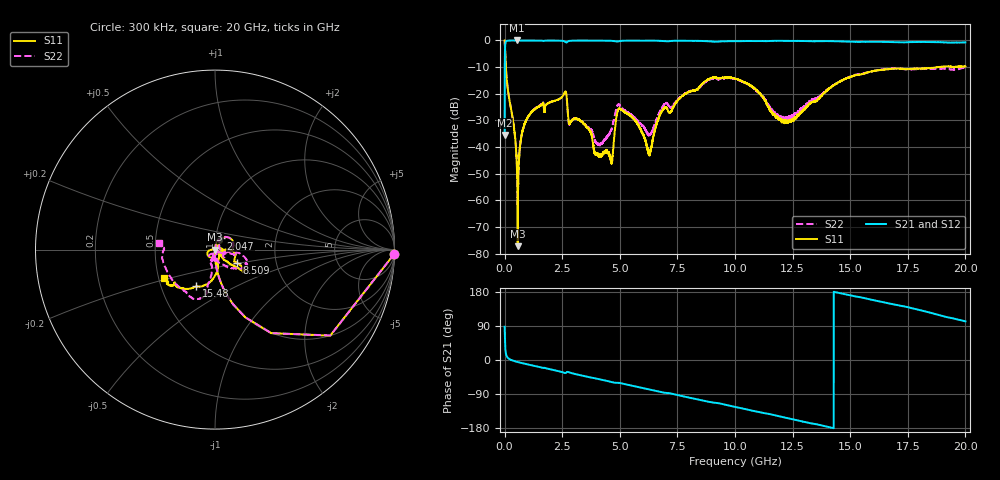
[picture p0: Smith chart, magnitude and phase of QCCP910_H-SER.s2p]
!{QCCP910}
!Johanson Technology Inc.
!www.johansontechnology.com
!Test Board Conditions:
!Substrate Type  RO4350B
!Substrate Thickness  20 mil
!Substrate Dk  3.66
!TL Type: GCPW
!TL Trace Width  36 mil
!TL Gap  12 mil
!Electrode orientation  Horizontal
!DUT TOPOLOGY	SERIES
!Mounting Pad LxW  26x36 mil
! Created Sat Jan  9 18:39:52 2021
# hz S ma R 50
! 2 Port Network Data from SP1.SP block
! freq  magS11  angS11  magS21  angS21  magS12  angS12  magS22  angS22
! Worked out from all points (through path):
!   20001 points, 300 kHz to 20 GHz, reference 50 ohm
!   highest |S21| = 0.00 dB at 527.3 MHz (marker M1); lowest = -35.5 dB at 300 kHz (marker M2)
!   group delay of S21, straight-line fit = 35.7 ps
!   lowest |S11| = -77.2 dB at 569.3 MHz (marker M3), VSWR 1.00, Z = 50 - j0.0123 ohm
!   |S11| at or under -10 dB: 53.16 MHz to 18.78 GHz (18.73 GHz wide, 199 % of centre); 18.80958 GHz to 18.8151 GHz (5.523 MHz wide, 0.0294 % of centre); 18.81673 GHz to 18.85819 GHz (41.46 MHz wide, 0.22 % of centre)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
!   |S22| runs from -61.7 to 0.0 dB; largest |S21 - S12| = 0.017
!   S11 on the Smith chart (normalised r, x): 300 kHz: 4, -81; 2.047 GHz: 1.06, +0.13; 8.509 GHz: 1.26, -0.19; 15.48 GHz: 0.75, -0.32; 20 GHz: 0.53, -0.19
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300000  0.9987 -1.4  0.0168 87.8  0.01695 88.5  0.9998 -1.3
1.093e8  0.1569 -81.8  0.9866 7.9  0.9868 7.9  0.1573 -81.8
5.273e8  0.005376 -96.4  0.9995 -4.6  0.9984 -4.6  0.005428 -86.0
5.693e8  0.000138 -116.5  0.9977 -5.4  0.9987 -5.3  0.0008788 -22.3
9.743e8  0.0342 79.3  0.9971 -11.3  0.9965 -11.2  0.03413 75.4
2.0473e9  0.07072 61.5  0.9939 -25.3  0.9935 -25.4  0.07107 66.9
2.6053e9  0.1051 37.6  0.959 -34.3  0.9594 -34.3  0.1035 38.3
2.8403e9  0.02821 32.9  0.9845 -33.3  0.9845 -33.3  0.02794 33.7
3.3343e9  0.0304 54.8  0.9942 -40.8  0.994 -40.8  0.03029 39.3
4.0683e9  0.00705 110.5  0.9927 -50.2  0.9929 -50.2  0.01143 -41.0
4.6003e9  0.006012 -165.5  0.9866 -57.5  0.9864 -57.5  0.02005 -77.1
4.9793e9  0.05267 -133.0  0.9699 -60.3  0.969 -60.3  0.06198 -115.9
5.7043e9  0.03025 -173.7  0.9925 -70.3  0.9924 -70.3  0.03321 -133.1
6.2693e9  0.007467 110.2  0.9914 -77.6  0.9917 -77.5  0.01718 -80.8
6.6673e9  0.03307 13.2  0.988 -83.1  0.9863 -83.0  0.03957 -26.5
8.5093e9  0.1421 -31.4  0.979 -105.7  0.9794 -105.7  0.1375 -8.2
1.00003e10  0.1929 -36.8  0.9704 -123.7  0.9691 -123.7  0.19 -32.3
1.20943e10  0.03182 -31.4  0.9834 -150.8  0.9855 -150.8  0.03584 -100.9
1.33343e10  0.06972 -80.0  0.9663 -167.5  0.968 -167.5  0.07741 -107.7
1.54793e10  0.2307 -117.4  0.9419 165.1  0.9452 164.9  0.2369 -102.0
1.66673e10  0.2889 -133.2  0.9355 149.5  0.9262 149.3  0.2969 -111.7
2e10  0.3261 -150.7  0.9209 101.9  0.9119 101.7  0.317 172.7
